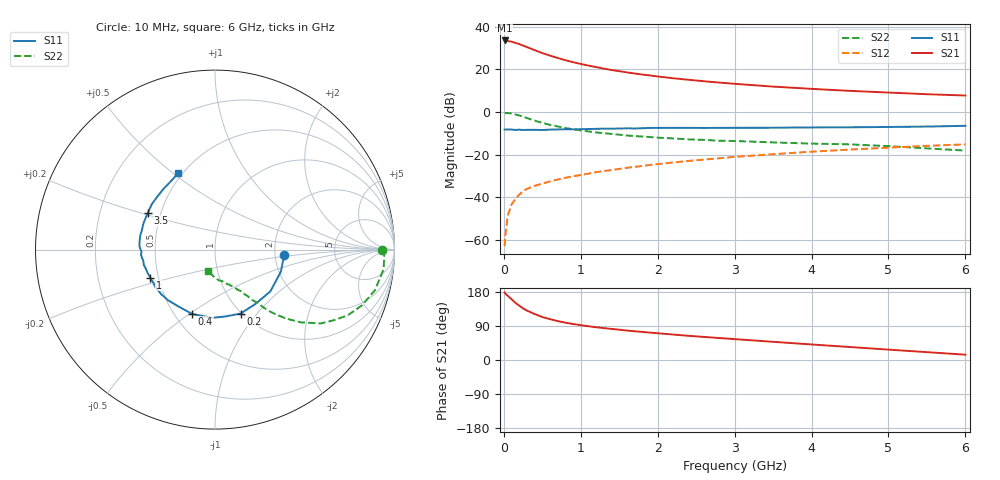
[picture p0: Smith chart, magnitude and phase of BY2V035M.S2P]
! SIEMENS Small Signal Semiconductors
! BFY420
! Si NPN RF SIEGET Grounded Emitter Transistor in MICRO-X
! VCE = 2 V  IC = 35 mA
! Common Emitter S-Parameters:  October  1996
# GHz  S  MA  R  50
!  f  S11  S21  S12  S22
! GHz  MAG  ANG  MAG  ANG  MAG  ANG  MAG  ANG
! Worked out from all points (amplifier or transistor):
!   36 points, 10 MHz to 6 GHz, reference 50 ohm
!   highest |S21| = 33.6 dB at 10 MHz (marker M1)
!   |S21| within 3 dB of that: start of sweep to 291.3 MHz
!   unconditionally stable (mu >= 1): start of sweep to 14.88 MHz; 1.428 GHz to end of sweep
!   at 250 MHz: K = 0.40, MSG = 34.3 dB, |S12| = -37.3 dB
!   at 1.4 GHz: K = 1.00, MSG = 23.5 dB, |S12| = -27.3 dB
!   at 6 GHz: K = 1.07, MAG = 9.9 dB, |S12| = -15.2 dB
!   S11 on the Smith chart (normalised r, x): 10 MHz: 2.25, -0.16; 200 MHz: 0.99, -0.83; 400 MHz: 0.61, -0.51; 1 GHz: 0.45, -0.17; 3.5 GHz: 0.42, +0.21; 6 GHz: 0.48, +0.52
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0.01  0.3872 -4.5  48 178.3  0.0007 122.7  0.9328 -0.1
0.02  0.3847 -8.0  47.73 175.2  0.0013 93.2  0.9432 -1.7
0.05  0.387 -18.6  46.47 169.5  0.0036 85.3  0.9459 -6.6
0.1  0.3864 -37.1  44.97 160.4  0.0067 77.4  0.9195 -14.2
0.15  0.3774 -53.6  42.18 150.8  0.009 72.9  0.8755 -20.8
0.2  0.3837 -68.2  39.51 143.5  0.0114 70.0  0.8259 -26.3
0.25  0.3771 -81.1  36.37 136.2  0.0136 66.7  0.7681 -30.9
0.3  0.3804 -92.3  33.5 130.4  0.0155 64.8  0.7207 -34.8
0.4  0.3807 -109.4  28.45 121.4  0.0183 63.2  0.6269 -40.3
0.5  0.3767 -122.8  24.2 113.4  0.0207 61.4  0.5552 -43.9
0.6  0.3847 -132.7  21.12 107.8  0.0233 60.6  0.4994 -46.6
0.7  0.3891 -140.1  18.6 102.7  0.0258 61.7  0.4565 -48.6
0.8  0.3923 -147.2  16.48 98.5  0.0283 61.3  0.4198 -50.1
1  0.3927 -156.6  13.44 92.0  0.0329 62.6  0.369 -52.1
1.1  0.3978 -161.4  12.33 89.0  0.0355 63.1  0.3488 -53.5
1.4  0.4043 -171.1  9.696 82.1  0.043 63.1  0.305 -55.9
1.6  0.4133 -176.2  8.514 77.7  0.0487 62.1  0.2803 -57.8
2.2  0.423 171.9  6.208 67.2  0.065 60.0  0.2393 -62.9
3.5  0.4261 151.4  3.947 48.0  0.1016 51.3  0.1927 -73.5
4.5  0.4364 137.4  3.133 34.2  0.1307 42.7  0.173 -82.4
5.5  0.454 122.4  2.614 20.7  0.1597 33.0  0.1393 -97.6
6  0.4725 115.8  2.437 14.0  0.173 28.0  0.1237 -108.7
